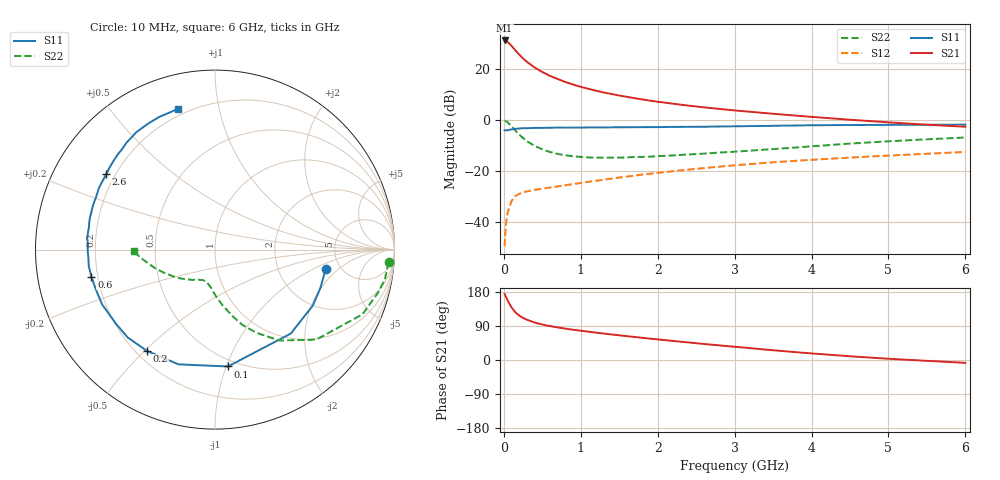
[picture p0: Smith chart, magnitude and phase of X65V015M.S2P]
! SIEMENS Small Signal Semiconductors
! BFP193W
! Si NPN RF Bipolar Junction Transistor in SOT343
! VCE = 5 V  IC = 15 mA
! Common Emitter S-Parameters:  April 1994
# GHz  S  MA  R  50
!  f  S11  S21  S12  S22
! GHz  MAG  ANG  MAG  ANG  MAG  ANG  MAG  ANG
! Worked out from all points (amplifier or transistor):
!   40 points, 10 MHz to 6 GHz, reference 50 ohm
!   highest |S21| = 31.1 dB at 10 MHz (marker M1)
!   |S21| within 3 dB of that: start of sweep to 125.4 MHz
!   unconditionally stable (mu >= 1): 1.141 GHz to 4.133 GHz
!   at 200 MHz: K = 0.29, MSG = 27.2 dB, |S12| = -28.9 dB
!   at 1.5 GHz: K = 1.09, MAG = 14.3 dB, |S12| = -22.5 dB
!   at 6 GHz: K = 0.93, MSG = 4.9 dB, |S12| = -12.5 dB
!   S11 on the Smith chart (normalised r, x): 10 MHz: 3.83, -1.37; 100 MHz: 0.44, -1.01; 200 MHz: 0.24, -0.51; 600 MHz: 0.18, -0.10; 2.6 GHz: 0.17, +0.30; 6 GHz: 0.17, +0.76
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0.01  0.6262 -10.0  35.87 174.2  0.0034 85.3  0.9695 -4.1
0.02  0.625 -19.9  35.69 170.2  0.0065 79.3  0.9608 -10.0
0.03  0.6279 -29.7  35.21 165.7  0.0099 78.2  0.9405 -14.6
0.05  0.6302 -47.9  33.54 156.7  0.0157 70.0  0.8974 -23.7
0.1  0.6552 -83.7  28.13 138.8  0.026 55.8  0.7545 -41.7
0.15  0.671 -107.7  23.01 125.9  0.0325 46.4  0.6203 -54.7
0.2  0.68 -123.9  18.94 117.2  0.0359 41.3  0.5169 -63.6
0.25  0.6901 -134.8  16.01 111.0  0.0385 38.3  0.4433 -70.3
0.3  0.6891 -143.0  13.69 106.2  0.0401 36.7  0.3843 -75.1
0.4  0.6993 -154.1  10.63 99.0  0.0429 35.5  0.3109 -82.5
0.5  0.7003 -162.1  8.66 93.6  0.0453 36.3  0.266 -88.0
0.6  0.7046 -167.7  7.272 89.5  0.0477 37.5  0.2364 -92.3
0.8  0.7069 -176.1  5.526 82.8  0.0528 40.6  0.2037 -98.5
1.1  0.7145 175.0  4.065 74.7  0.0617 44.6  0.1847 -105.8
1.3  0.7131 170.1  3.446 69.7  0.068 46.6  0.1832 -109.5
1.6  0.7197 163.5  2.83 62.8  0.0781 48.7  0.1851 -114.1
2.2  0.7319 152.3  2.078 50.3  0.0995 50.0  0.2023 -124.0
2.6  0.7371 145.3  1.766 42.3  0.1143 49.7  0.2191 -130.5
3.2  0.7581 135.6  1.447 31.3  0.1369 47.7  0.2514 -140.3
4.5  0.7949 117.9  1.01 9.8  0.1835 41.0  0.3451 -161.8
5.5  0.8037 108.9  0.807 -2.2  0.2183 35.4  0.4182 -174.0
6  0.8108 104.7  0.737 -7.5  0.2368 32.9  0.4532 -178.8
